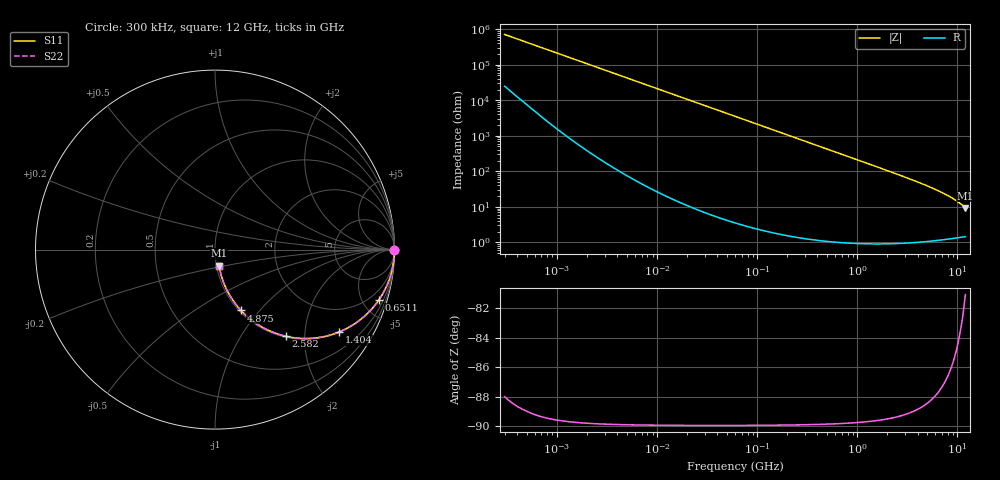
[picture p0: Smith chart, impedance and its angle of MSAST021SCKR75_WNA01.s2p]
! MSAST021SCKR75_WNA01  S-PARAMETER MODEL  ( General Type )
! Model Generated by TAIYO YUDEN Corporation (http://www.ty-top.com)
! Version 2.0
! TAIYO YUDEN Control No. 181101
! Copyright(c) 2015 TAIYO YUDEN CO.,LTD. All Rights Reserved.
! Product Description (link to TY-COMPAS)
! https://ds.yuden.co.jp/TYCOMPAS/or/detail?pn=MSAST021SCKR75BWNA01&u=M
! Products Name : Multilayer Ceramic Capacitors
! Characteristics :
!  Capacitance : 0.75 pF , Rated Voltage : 25V , TCC : CK / C0K
!  Case Size : 0.25 x 0.125 / 0.0098 x 0.0049 [mm/inch] , Thickness : 0.125 / 0.0049 [mm/inch]
!  (Conditions: Temperature = 25 degC , DC Bias Current/Voltage = 0A / 0V)
! External Node Assignments :
!  1  o---| |---o  2
! GND o---------o GND
! Frequency Range : 0.3MHz  -  12000MHz  [ 401 STEP ]
# MHz S RI R 50
! Freq[MHz].  S11 Real  S11 Imag  S21 Real  S21 Imag  S12 Real  S12 Imag  S22 Real  S22 Imag
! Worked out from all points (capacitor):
!   401 points, 300 kHz to 12 GHz, reference 50 ohm
!   read as one part in series: C = 750 fF near 316.3 kHz
!   lowest |Z| = 9.31 ohm at 12 GHz (marker M1)
!   S11 on the Smith chart (normalised r, x): 300 kHz: open; 651.1 MHz: 1.02, -6.51; 1.404 GHz: 1.02, -3.00; 2.582 GHz: 1.02, -1.61; 4.875 GHz: 1.02, -0.80; 12 GHz: 1.03, -0.18
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0.3  1 -0.000141  4.97e-06 0.000141  4.97e-06 0.000141  1 -0.000141
0.316324  1 -0.000149  4.87e-06 0.000149  4.87e-06 0.000149  1 -0.000149
1.769972  1 -0.000834  4.04e-06 0.000834  4.04e-06 0.000834  1 -0.000834
10.44266  1 -0.00492  3.03e-05 0.00492  3.03e-05 0.00492  1 -0.00492
60  0.9992 -0.0283  0.000827 0.0283  0.000827 0.0283  0.9992 -0.0283
164.1901  0.9939 -0.0769  0.00605 0.0769  0.00605 0.0769  0.9939 -0.0769
244.3004  0.9867 -0.1136  0.0133 0.1136  0.0133 0.1136  0.9867 -0.1136
353.9943  0.9726 -0.1623  0.0274 0.1623  0.0274 0.1623  0.9726 -0.1623
486.4723  0.9495 -0.2177  0.0505 0.2177  0.0505 0.2177  0.9495 -0.2177
651.0506  0.913 -0.2802  0.087 0.2802  0.087 0.2802  0.913 -0.2802
968.706  0.8256 -0.3773  0.1744 0.3773  0.1744 0.3773  0.8256 -0.3773
1403.667  0.6918 -0.4587  0.3082 0.4587  0.3082 0.4587  0.6918 -0.4587
1735.023  0.5938 -0.4874  0.4062 0.4874  0.4062 0.4874  0.5938 -0.4874
2088.533  0.5007 -0.4954  0.4993 0.4954  0.4993 0.4954  0.5007 -0.4954
2581.562  0.3937 -0.4828  0.6063 0.4828  0.6063 0.4828  0.3937 -0.4828
3547.679  0.2509 -0.4251  0.7491 0.4251  0.7491 0.4251  0.2509 -0.4251
4875.354  0.1449 -0.3391  0.8551 0.3391  0.8551 0.3391  0.1449 -0.3391
6354.153  0.0859 -0.2612  0.9141 0.2612  0.9141 0.2612  0.0859 -0.2612
8064.993  0.0516 -0.193  0.9484 0.193  0.9484 0.193  0.0516 -0.193
9708.23  0.0343 -0.1428  0.9657 0.1428  0.9657 0.1428  0.0343 -0.1428
11380.75  0.0246 -0.1019  0.9754 0.1019  0.9754 0.1019  0.0246 -0.1019
12000  0.0223 -0.0886  0.9777 0.0886  0.9777 0.0886  0.0223 -0.0886
